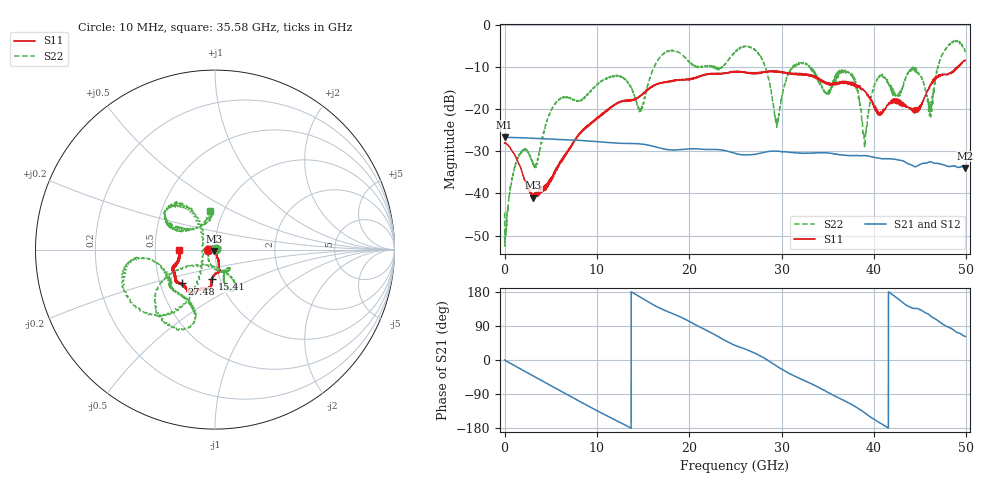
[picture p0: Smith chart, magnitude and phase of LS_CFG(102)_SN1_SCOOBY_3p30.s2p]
!Keysight Technologies,N5245B,MY58422026,A.13.80.08
!Date: Thursday, March 19, 2020 23:59:08
!Correction: S11(Full 2 Port(1,2))
!S21(Full 2 Port(1,2))
!S12(Full 2 Port(1,2))
!S22(Full 2 Port(1,2))
!S2P File: Measurements: S11, S21, S12, S22:
# Hz S DB R 50.0
!freq dBS11 angS11 dBS21 angS21 dBS12 angS12 dBS22 angS22
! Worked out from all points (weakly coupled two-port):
!   4991 points, 10 MHz to 49.91 GHz, reference 50 ohm
!   highest |S21| = -26.67 dB at 10 MHz (marker M1); lowest = -33.9 dB at 49.91 GHz (marker M2)
!   lowest |S11| = -41.0 dB at 3.11 GHz (marker M3), VSWR 1.02, Z = 49.5 - j0.739 ohm
!   |S11| at or under -10 dB: start of sweep to 49.01 GHz; 49.04996 GHz to 49.1085 GHz (58.54 MHz wide, 0.119 % of centre); 49.18892 GHz to 49.20766 GHz (18.74 MHz wide, 0.0381 % of centre)
!   |S22| runs from -52.5 to -3.7 dB; largest |S21 - S12| = 0.00044
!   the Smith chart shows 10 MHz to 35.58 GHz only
!   S11 on the Smith chart (normalised r, x): 10 MHz: 0.92, -0.00; 15.41 GHz: 0.92, -0.31; 27.48 GHz: 0.65, -0.26; 35.58 GHz: 0.66, -0.01
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1e7  -28.02 -176.1  -26.67 -0.3  -26.67 -0.3  -44.55 9.2
1.49e9  -32.74 -175.4  -26.78 -20.3  -26.77 -20.3  -31.11 -6.7
3.11e9  -41.01 -123.0  -26.91 -42.1  -26.90 -42.1  -33.08 100.5
5.51e9  -34.42 -71.3  -27.16 -74.6  -27.15 -74.5  -18.61 -84.0
8.33e9  -25.58 -72.9  -27.45 -111.8  -27.45 -111.8  -17.83 -62.3
1.541e10  -15.61 -95.0  -28.48 155.7  -28.47 155.8  -15.29 -146.2
1.665e10  -14.03 -96.5  -29.14 138.9  -29.13 139.0  -8.24 -145.3
1.985e10  -12.93 -103.7  -29.47 104.0  -29.47 104.1  -8.57 -106.5
2.496e10  -11.19 -123.1  -30.47 38.6  -30.46 38.9  -6.54 -171.1
2.748e10  -11.55 -134.6  -30.60 13.7  -30.60 14.0  -6.73 -128.0
2.947e10  -10.98 -140.9  -29.98 -16.1  -29.97 -15.7  -23.46 -176.8
3.103e10  -11.51 -148.3  -30.30 -37.9  -30.31 -37.7  -10.40 125.5
3.328e10  -12.08 -159.0  -30.42 -63.7  -30.43 -63.2  -10.65 153.0
3.558e10  -13.82 -178.2  -30.60 -92.7  -30.54 -92.2  -13.43 99.8
3.759e10  -14.18 170.5  -31.02 -117.5  -30.96 -117.4  -12.21 127.7
3.902e10  -15.72 168.8  -31.02 -139.6  -31.01 -139.8  -28.20 -113.1
4.021e10  -20.45 154.9  -31.52 -159.5  -31.50 -159.6  -13.46 -9.1
4.16e10  -18.59 103.9  -31.79 179.6  -31.82 179.7  -14.19 22.3
4.445e10  -20.19 53.3  -33.69 136.1  -33.70 136.4  -10.42 -17.1
4.614e10  -14.24 8.5  -32.51 116.3  -32.54 116.4  -21.55 -51.1
4.757e10  -11.72 7.3  -33.28 93.0  -33.28 93.1  -6.29 -80.3
4.991e10  -8.45 -12.8  -33.95 62.3  -33.97 62.5  -6.28 -28.6
